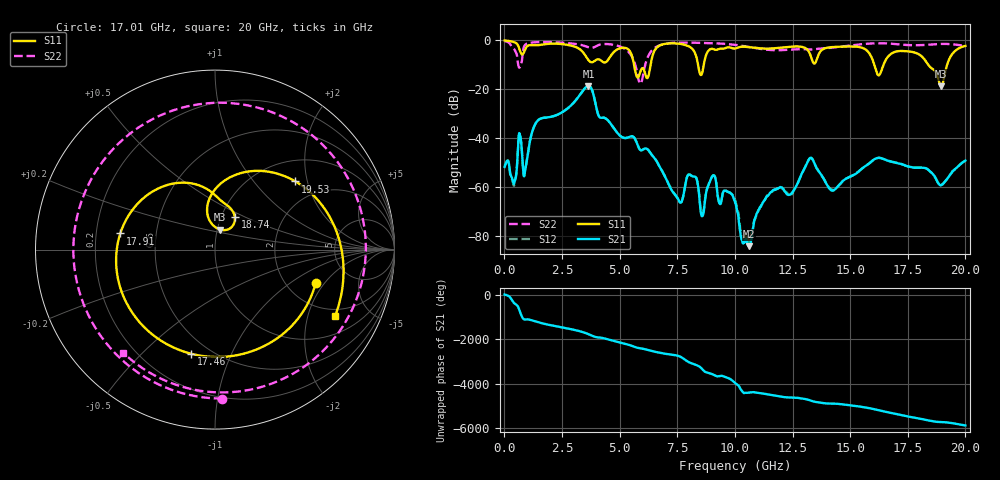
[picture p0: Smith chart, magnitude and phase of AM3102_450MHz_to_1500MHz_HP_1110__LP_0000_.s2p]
!Agilent Technologies,E8364B,MY43040894,A.07.50.67
!Agilent E8364B: A.07.50.67
!Date: Thursday, January 11, 2018 06:42:00
!Correction: S11(Full 2 Port(1,2))
!S21(Full 2 Port(1,2))
!S12(Full 2 Port(1,2))
!S22(Full 2 Port(1,2))
!S2P File: Measurements: S11, S21, S12, S22:
# Hz S  dB  R 50
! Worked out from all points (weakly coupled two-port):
!   1601 points, 10 MHz to 20 GHz, reference 50 ohm
!   highest |S21| = -18.67 dB at 3.646 GHz (marker M1); lowest = -84.1 dB at 10.59 GHz (marker M2)
!   lowest |S11| = -18.8 dB at 18.95 GHz (marker M3), VSWR 1.26, Z = 51.6 + j11.7 ohm
!   |S11| at or under -10 dB: 5.624 GHz to 6.344 GHz (720.1 MHz wide, 12 % of centre); 16.05 GHz to 16.45 GHz (401.3 MHz wide, 2.47 % of centre); 18.39 GHz to 19.21 GHz (823 MHz wide, 4.38 % of centre)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
!   |S22| runs from -17.7 to -0.3 dB; largest |S21 - S12| = 0.00032
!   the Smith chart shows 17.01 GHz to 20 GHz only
!   S11 on the Smith chart (normalised r, x): 17.01 GHz: 2.85, -1.64; 17.46 GHz: 0.40, -0.71; 17.91 GHz: 0.30, +0.08; 18.74 GHz: 1.16, +0.44; 19.53 GHz: 1.46, +1.69; 20 GHz: 1.68, -3.00
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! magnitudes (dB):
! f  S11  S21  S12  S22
! 10 MHz  -0.1  -51.7  -51.2  -0.3
! 409.8 MHz  -0.8  -58.6  -59.4  -3.5
! 3.346 GHz  -4.2  -21.4  -21.4  -2.0
! 3.646 GHz  -8.1  -18.7  -18.7  -2.9
! 5.895 GHz  -13.0  -44.8  -44.8  -17.7
! 6.682 GHz  -2.5  -50.7  -50.8  -2.3
! 7.606 GHz  -1.5  -66.2  -65.7  -1.0
! 8.081 GHz  -2.9  -55.1  -55.1  -1.0
! 8.531 GHz  -14.2  -70.7  -70.0  -1.1
! 9.055 GHz  -3.6  -55.2  -55.2  -1.2
! 10.01 GHz  -3.4  -66.1  -65.2  -1.9
! 10.59 GHz  -2.8  -84.1  -81.4  -2.7
! 13.34 GHz  -7.8  -48.3  -48.3  -3.8
! 14.24 GHz  -2.8  -61.4  -61.2  -3.0
! 16.68 GHz  -6.4  -49.3  -49.3  -1.4
! 17.01 GHz  -4.6  -50.1  -50.1  -1.6
! 17.46 GHz  -4.5  -51.4  -51.4  -2.0
! 17.91 GHz  -5.4  -52.1  -52.0  -2.0
! 18.74 GHz  -13.5  -56.8  -56.9  -1.6
! 18.95 GHz  -18.8  -59.2  -59.2  -1.5
! 19.53 GHz  -4.6  -52.9  -52.8  -1.7
! 20 GHz  -2.3  -49.1  -49.2  -2.3
